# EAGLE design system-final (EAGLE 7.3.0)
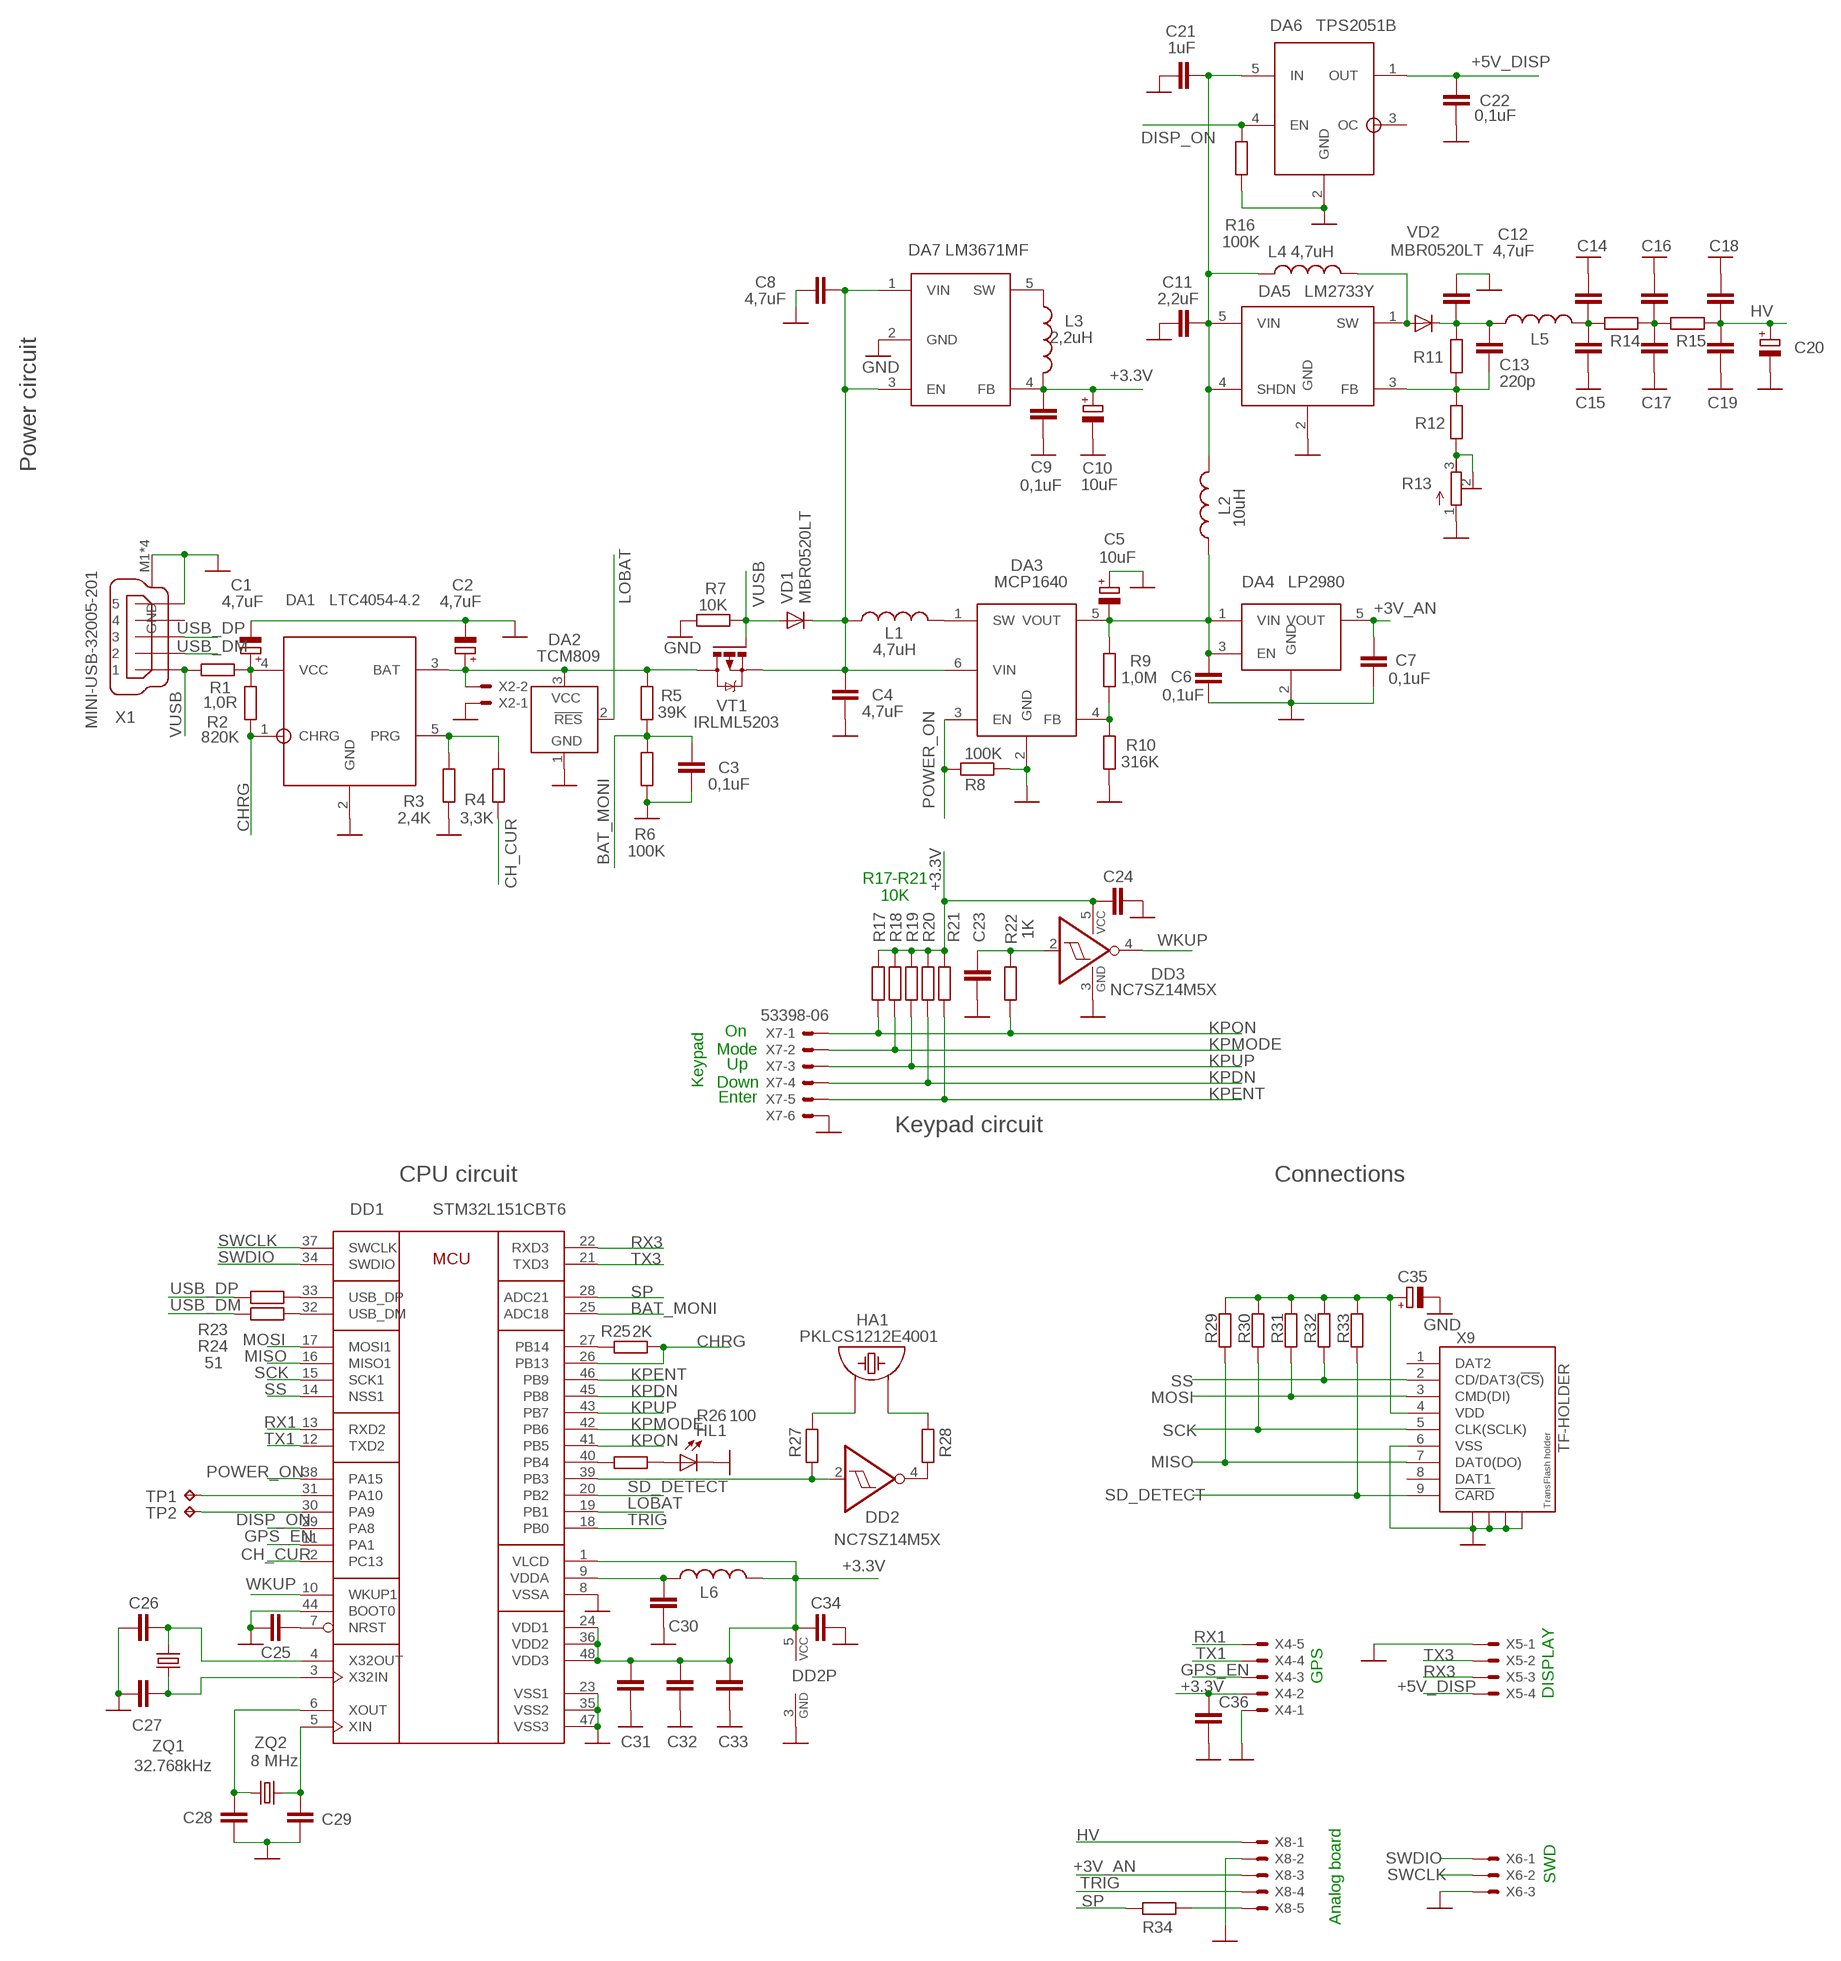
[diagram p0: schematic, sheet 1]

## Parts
C1  4,7uF  CPOL-EUSMCA  [SMC_A]
C2  4,7uF  CPOL-EUSMCA  [SMC_A]
C3  0,1uF  C-EUC0603  [C0603]
C4  4,7uF  C-EUC0805  [C0805]
C5  10uF  CPOL-EUSMCB  [SMC_B]
C6  0,1uF  C-EUC0603  [C0603]
C7  0,1uF  C-EUC0603  [C0603]
C8  4,7uF  C-EUC1206  [C1206]
C9  0,1uF  C-EUC1206  [C1206]
C10  10uF  CPOL-EUSMCB  [SMC_B]
C11  2,2uF  C-EUC0805  [C0805]
C12  4,7uF  C-EUC1206  [C1206]
C13  220p  C-EUC0603  [C0603]
C14  C-EUC0603  [C0603]
C15  C-EUC0603  [C0603]
C16  C-EUC0603  [C0603]
C17  C-EUC0603  [C0603]
C18  C-EUC0603  [C0603]
C19  C-EUC0603  [C0603]
C20  CPOL-EUSMCE  [SMC_E]
C21  1uF  C-EUC0805  [C0805]
C22  0,1uF  C-EUC0805  [C0805]
C23  C-EUC0603  [C0603]
C24  C-EUC0603  [C0603]
C25  C-EUC0603  [C0603]
C26  C-EUC0603  [C0603]
C27  C-EUC0603  [C0603]
C28  C-EUC0603  [C0603]
C29  C-EUC0603  [C0603]
C30  C-EUC0603  [C0603]
C31  C-EUC0603  [C0603]
C32  C-EUC0603  [C0603]
C33  C-EUC0603  [C0603]
C34  C-EUC0603  [C0603]
C35  CPOL-EUSMCA  [SMC_A]
C36  C-EUC0805  [C0805]
DA1  LTC4054-4.2  [SOT23-5L]
DA2  TCM809  [SOT23B-3]
DA3  MCP1640  [SOT23-6]
DA4  LP2980  [SOT23-5L]
DA5  LM2731Y  [SOT23-5L]
DA6  TPS2051B  [SOT23-5L]
DA7  LM3671  [SOT23-5]
DD1  STM32L151CBT6  STM32L151C  [LQFP48]
DD2  NC7SZ14M5X  [SOT23-5]
DD3  NC7SZ14M5X  [SOT23-5]
HA1  PKLCS1212E4001  [PKLCS1212E4001]
HL1  LEDCHIP-LED0805  [CHIP-LED0805]
L1  4,7uH  L-USL1812  [L1812]
L2  10uH  L-USL2825P  [L2825P]
L3  2,2uH  L-USL2825P  [L2825P]
L4  4,7uH  L-USL1812  [L1812]
L5  L-USL2825P  [L2825P]
L6  L-USL3225M  [L3225M]
R1  1,0R  R-EU_M1206  [M1206]
R2  820K  R-EU_R0603  [R0603]
R3  2,4K  R-EU_R0603  [R0603]
R4  3,3K  R-EU_R0603  [R0603]
R5  39K  R-EU_R0603  [R0603]
R6  100K  R-EU_R0603  [R0603]
R7  10K  R-EU_R0603  [R0603]
R8  100K  R-EU_R0603  [R0603]
R9  1,0M  R-EU_R0603  [R0603]
R10  316K  R-EU_R0603  [R0603]
R11  R-EU_R0603  [R0603]
R12  R-EU_R0603  [R0603]
R13  R-TRIMM3103  [RTRIM3103]
R14  R-EU_R0603  [R0603]
R15  R-EU_R0603  [R0603]
R16  100K  R-EU_R0603  [R0603]
R17  10K  R-EU_R0603  [R0603]
R18  10K  R-EU_R0603  [R0603]
R19  10K  R-EU_R0603  [R0603]
R20  10K  R-EU_R0603  [R0603]
R21  10K  R-EU_R0603  [R0603]
R22  1K  R-EU_R0603  [R0603]
R23  51  R-EU_R0603  [R0603]
R24  51  R-EU_R0603  [R0603]
R25  2K  R-EU_R0603  [R0603]
R26  100  R-EU_R0603  [R0603]
R27  R-EU_R0603  [R0603]
R28  R-EU_R0603  [R0603]
R29  R-EU_R0603  [R0603]
R30  R-EU_R0603  [R0603]
R31  R-EU_R0603  [R0603]
R32  R-EU_R0603  [R0603]
R33  R-EU_R0603  [R0603]
R34  R-EU_R0603  [R0603]
TP1  TPB1,27  [B1,27]
TP2  TPB1,27  [B1,27]
VD1  MBR0520LT  [SOD123]
VD2  MBR0520LT  [SOD123]
VT1  IRLML5203  [MICRO3]
X1  MINI-USB-32005-201  [32005-201]
X2  53398-02  [53398-02]
X4  53398-05  [53398-05]
X5  53398-04  [53398-04]
X6  53398-03  [53398-03]
X7  53398-06  [53398-06]
X8  53398-05  [53398-05]
X9  TF-HOLDER  [TF-PULL]
ZQ1  32.768kHz  CRYSTAL-32.768KHZPTH-2X6-KIT  [CRYSTAL-PTH-2X6-CYL-KIT]
ZQ2  CRYSTALPTH-HC49US  [HC49US]

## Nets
5V_D: C11.2 C21.2 DA5.4(SHDN) DA5.5(VIN) DA6.5(IN) L2.2 L4.1
+3.3V: C9.2 C10.+ C24.1 C31.1 C32.1 C33.1 C34.1 C35.+ C36.1 DA7.4(FB) DD1.1(VLCD) DD1.24(VDD1) DD1.36(VDD2) DD1.48(VDD3) DD2.5(VCC) DD3.5(VCC) L3.2 L6.2 R17.2 R18.2 R19.2 R20.2 R21.2 R29.2 R30.2 R31.2 R32.2 R33.2 X4.2 X9.4(VDD)
+3V_AN: C7.1 DA4.5(VOUT) X8.3
+5V_DIRT: C5.- C6.1 DA3.5(VOUT) DA4.1(VIN) DA4.3(EN) L2.1 R9.2
+5V_DISP: C22.1 DA6.1(OUT) X5.4
BAT_MONI: C3.1 DD1.25(ADC18) R5.1 R6.2
BUZ: DD1.39(PB3) DD2.2(I) R27.1
CH_CUR: DD1.2(PC13) R4.1
CHRG: DA1.1(CHRG) DD1.26(PB13) R2.1 R25.1
DISP_ON: DA6.4(EN) DD1.29(PA8) R16.2
GND: C1.- C2.- C3.2 C4.2 C5.+ C6.2 C7.2 C8.1 C9.1 C10.- C11.1 C12.1 C14.1 C15.2 C16.1 C17.2 C18.1 C19.2 C20.- C21.1 C22.2 C23.2 C24.2 C25.2 C26.1 C27.1 C28.2 C29.2 C30.1 C31.2 C32.2 C33.2 C34.2 C35.- C36.2 DA1.2(GND) DA2.1(GND) DA3.2(GND) DA4.2(GND) DA5.2(GND) DA6.2(GND) DA7.2(GND) DD1.8(VSSA) DD1.23(VSS1) DD1.35(VSS2) DD1.44(BOOT0) DD1.47(VSS3) DD2.3(GND) DD3.3(GND) HL1.C R3.1 R6.1 R7.1 R8.1 R10.1 R13.1(A) R16.1 X1.5 X1.M1(GND) X1.M2(GND) X1.M3(GND) X1.M4(GND) X2.1 X4.1 X5.1 X6.3 X7.6 X8.2 X9.6(VSS) X9.S1 X9.S2 X9.S3 X9.S4
GPS_EN: DD1.11(PA1) X4.3
HV: C18.2 C19.1 C20.+ R15.2 X8.1
KPDN: DD1.45(PB8) R20.1 X7.4
KPENT: DD1.46(PB9) R21.1 X7.5
KPMODE: DD1.42(PB6) R18.1 X7.2
KPON: DD1.41(PB5) R17.1 R22.2 X7.1
KPUP: DD1.43(PB7) R19.1 X7.3
LED: DD1.40(PB4) R26.2
LOBAT: DA2.2(!RES) DD1.19(PB1)
MISO: DD1.16(MISO1) R29.1 X9.7(DAT0(DO))
MOSI: DD1.17(MOSI1) R31.1 X9.3(CMD(DI))
N$1: DD1.31(PA10) TP1.TP
N$2: C25.1 DD1.7(NRST)
N$3: C1.+ DA1.4(VCC) R1.2 R2.2
N$5: DA3.1(SW) L1.2
N$6: DA5.1(SW) L4.2 VD2.A
N$7: DA3.4(FB) R9.1 R10.2
N$8: C13.2 DA5.3(FB) R11.1 R12.2
N$9: C12.2 C13.1 L5.1 R11.2 VD2.C
N$10: R12.1 R13.2(S) R13.3(E)
N$11: C28.1 DD1.6(XOUT) ZQ2.1
N$12: C14.2 C15.1 L5.2 R14.1
N$13: C16.2 C17.1 R14.2 R15.1
N$14: C27.2 DD1.3(X32IN) ZQ1.2
N$15: C26.2 DD1.4(X32OUT) ZQ1.1
N$16: C29.1 DD1.5(XIN) ZQ2.2
N$18: DD1.30(PA9) TP2.TP
N$19: DD2.4(O) R28.1
N$20: HA1.P$2 R27.2
N$21: HA1.P$1 R28.2
N$23: HL1.A R26.1
N$24: DA7.5(SW) L3.1
N$25: DD1.27(PB14) R25.2
N$26: C23.1 DD3.2(I) R22.1
N$27: DD1.33(USB_DP) R23.1
N$28: DD1.32(USB_DM) R24.1
N$30: DA1.5(PRG) R3.2 R4.2
POWER_ON: DA3.3(EN) DD1.38(PA15) R8.2
RX1: DD1.13(RXD2) X4.5
RX3: DD1.22(RXD3) X5.3
SCK: DD1.15(SCK1) R30.1 X9.5(CLK(SCLK))
SD_DETECT: DD1.20(PB2) R33.1 X9.9(!CARD)
SP: DD1.28(ADC21) R34.2
SP_IN: R34.1 X8.5
SS: DD1.14(NSS1) R32.1 X9.2(CD/DAT3(!CS!))
SWCLK: DD1.37(SWCLK) X6.2
SWDIO: DD1.34(SWDIO) X6.1
TRIG: DD1.18(PB0) X8.4
TX1: DD1.12(TXD2) X4.4
TX3: DD1.21(TXD3) X5.2
USB_DM: R24.2 X1.2
USB_DP: R23.2 X1.3
VBAT: C2.+ DA1.3(BAT) DA2.3(VCC) R5.2 VT1.3(D) X2.2
VDDA: C30.2 DD1.9(VDDA) L6.1
VMASTER: C4.1 C8.2 DA3.6(VIN) DA7.1(VIN) DA7.3(EN) L1.1 VD1.C VT1.2(S)
VUSB: R1.1 R7.2 VD1.A VT1.1(G) X1.1
WKUP: DD1.10(WKUP1) DD3.4(O)
Unconnected: DA6.3(OC) X1.4 X9.1(DAT2) X9.8(DAT1)

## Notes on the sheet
- DA6   TPS2051B
- DA7 LM3671MF
- DA5   LM2733Y
- Power circuit
- DA3
- DA4   LP2980
- DA1   LTC4054-4.2
- TCM809
- R17-R21
  10K
- On
- Mode
- Up
- Keypad | Down
- Enter
- Keypad circuit
- CPU circuit | Connections
- GPS
- DISPLAY
- 8 MHz
- SWD
- Analog board

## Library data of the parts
C1 C2 C5 C10 C20 C35 = resistor:CPOL-EU: POLARIZED CAPACITOR, European symbol
C3 C4 C6-C9 C11-C19 C21-C34 C36 = resistor:C-EU: CAPACITOR, European symbol
DA1 = LTC4054-4.2:LTC4054-4.2
DA2 = telcom:TCM809: POWER SUPPLY MONITOR replacement for Maxim MAX809 and MAX810; MF: MICROCHIP; MPN: TCM809MENB713; OC_FARNELL: 9762744; OC_NEWARK: 96K3998
DA3 = MCP1640:MCP1640; MPN: MCP1640
DA4 = LP2980:LP2980
DA5 = LM2731Y:LM2731Y
DA6 = TPS2051B:TPS2051B: CURRENT-LIMITED, POWER-DISTRIBUTION SWITCH
DA7 = LM3671MF:LM3671
DD1 = stm32L151C:STM32L151C
DD2 DD3 = 74xx-little-de:NC7SZ14: TinyLogic(R) UHS Inverter with Schmitt Trigger Input Source: http://www.fairchildsemi.com/ds/NC/NC7SZ14.pdf
HA1 = PKLCS1212E:PKLCS1212E4001: SMD piezoelectric buzzer 12x12x3 mm, Murata
HL1 = adafruit:LED: LED
L1-L6 = resistor:L-US: INDUCTOR, American symbol
R1-R12 R14-R34 = resistor:R-EU_: RESISTOR, European symbol
R13 = resistor:R-TRIMM: Trimm resistor
TP1 TP2 = testpad:TP: Test pad
VD1 VD2 = diode:MBR0520LT: SCHOTTKY BARRIER RECTIFIER
VT1 = transistor-power:IRLML5203: HEXFET P-Channel Power MOSFET
X1 = con-cypressindustries:MINI-USB-: MINI USB-B Conector Source: www.cypressindustries.com; OC_FARNELL: unknown; OC_NEWARK: unknown
X2 = con-molex:53?-02: CONNECTOR; OC_FARNELL: unknown; OC_NEWARK: unknown
X4 X8 = con-molex:53?-05: CONNECTOR wire to board 1.25 mm (.049 inch) pitch header; OC_FARNELL: 1125354; OC_NEWARK: unknown
X5 = con-molex:53?-04: CONNECTOR wire to board 1.25 mm (.049 inch) pitch header; OC_FARNELL: 1125367; OC_NEWARK: unknown
X6 = con-molex:53?-03: CONNECTOR wire to board 1.25 mm (.049 inch) pitch header; OC_FARNELL: unknown; OC_NEWARK: unknown
X7 = con-molex:53?-06: CONNECTOR wire to board 1.25 mm (.049 inch) pitch header; OC_FARNELL: 1125368; OC_NEWARK: unknown
X9 = sd-mmc:TF-HOLDER: TF / Micro SD socket is PUSH-PUSH type, the card can be pushed into and auto locked and pushed out by simply press the card. Surface Mounting type.
ZQ1 = SparkFun-Clocks:CRYSTAL-32.768KHZ: 32.768kHz Crystal; PROD_ID: XTAL-10112
ZQ2 = SparkFun-Clocks:CRYSTAL: Crystals (Generic)

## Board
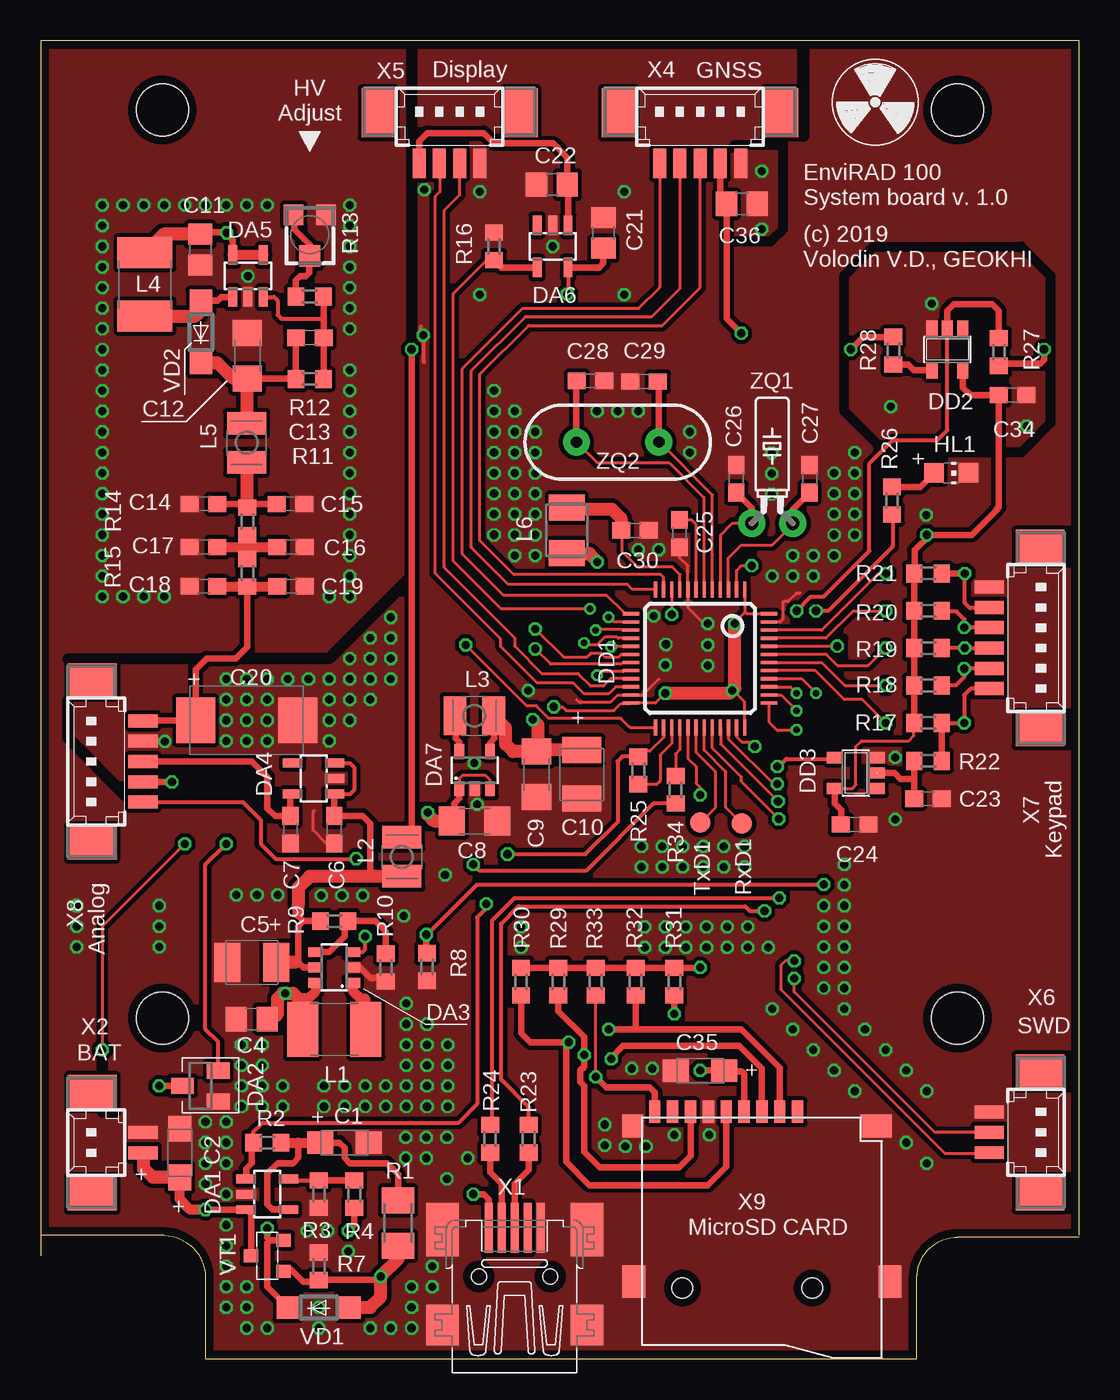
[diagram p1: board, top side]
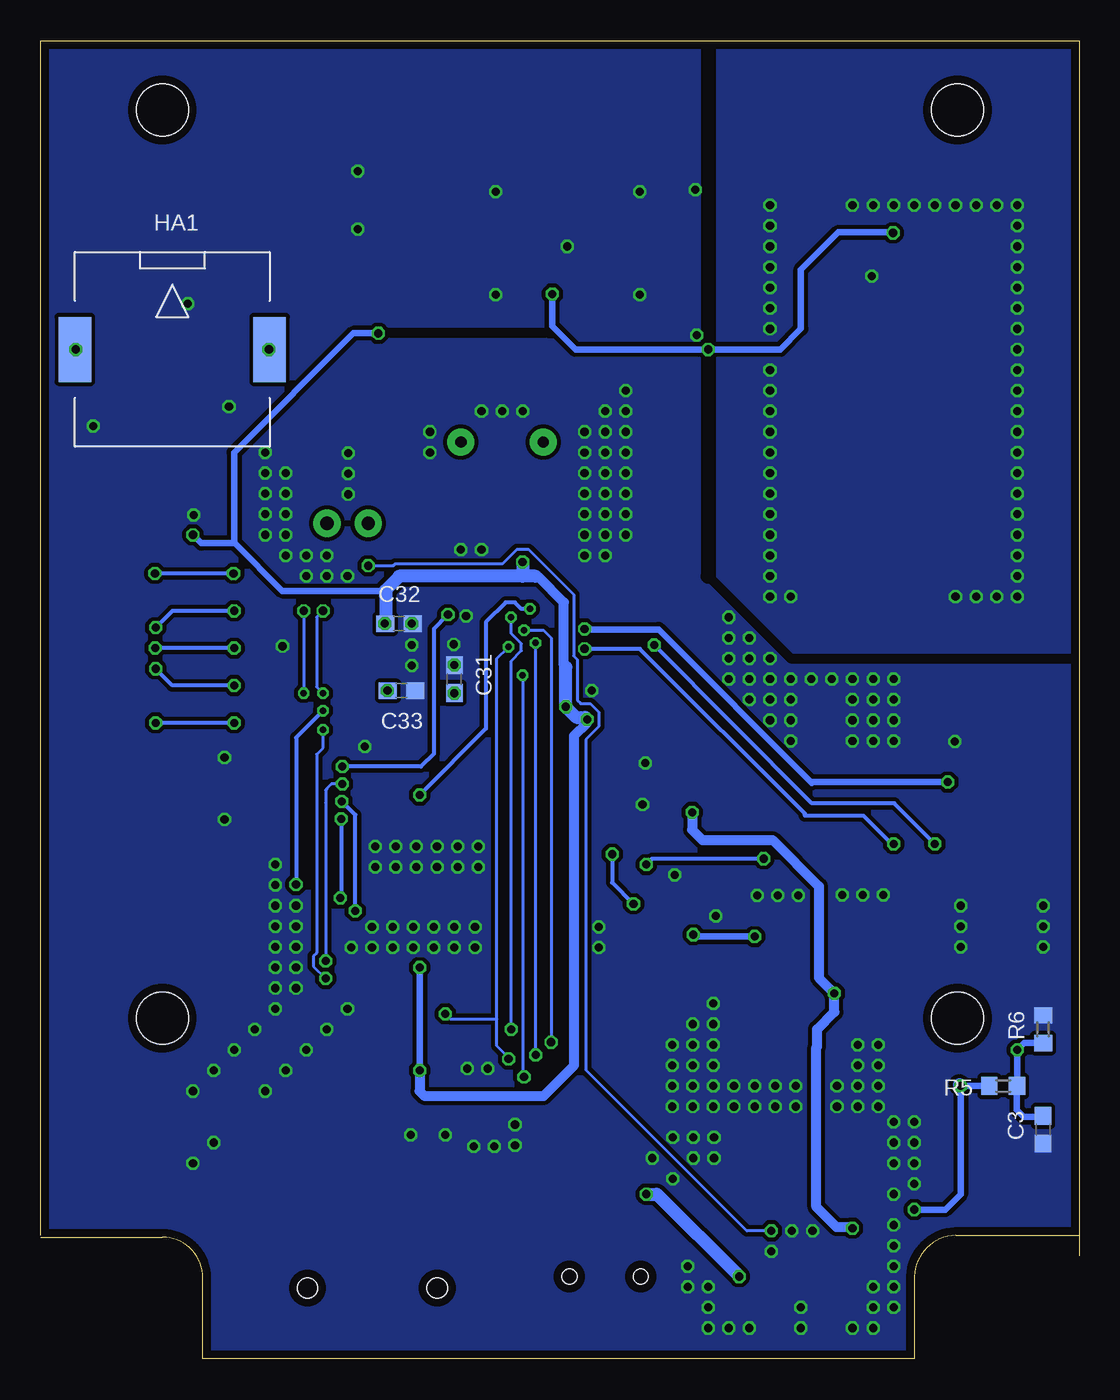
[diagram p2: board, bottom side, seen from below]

Size 64 x 81.27 mm. Coordinates in mm from the lower left corner, seen from the top.
Outline: 53.98,0 10.16,0 10.16,5.08 arc86 7.62,7.62 0,7.62
Outline: 64,7.62 64,81.27 0,81.27 0,7.62
Outline: 54,0 54,5 arc-90 56.5,7.5 64,7.5
Outline: 0,7.62 0,6.35
Copper layers (1*16): Top 0.035mm / dielectric 1.6mm / Bottom 0.035mm
Design rules "Elecrow_2-layer_PCB_eagle_rule": minimum track width 6mil, minimum drill 12mil, track to track 6mil, track to pad 6mil, pad to pad 6mil, via to via 8mil, smd to smd 0mil, copper to edge 20mil, drill to drill 10mil, minimum pad ring 6mil, minimum via ring 6mil, stop-mask expansion 0mil, vias tented up to drill 100mil, thermal gap 10mil
Holes 3.2 mm at 56.5,21 7.5,21 56.5,76.98 7.5,76.98
tRestrict: area 43.2,37.1 to 44.8,38.4; area 48.3,43.2 to 49.5,44.5; 25 lines
bRestrict: 7 lines

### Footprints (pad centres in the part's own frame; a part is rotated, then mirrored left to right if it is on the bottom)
SMC_A = smd 1.6 x 1.4: + -1.5,0; - 1.5,0
C0603 = smd 1.1 x 1: 1 -0.85,0; 2 0.85,0
C0805 = smd 1.3 x 1.5: 1 -0.95,0; 2 0.95,0
SMC_B = smd 1.6 x 2.4: + -1.5,0; - 1.5,0
C1206 = smd 1.6 x 1.8: 1 -1.4,0; 2 1.4,0
SMC_E = smd 2.4 x 2.8: + -3.15,0; - 3.15,0
SOT23-5L = smd 0.55 x 1.2: 1 -0.95,-1.3; 2 0,-1.3; 3 0.95,-1.3; 4 0.95,1.3; 5 -0.95,1.3
SOT23B-3 = smd 1 x 1.4: 1 -0.95,-1.1; 2 0.95,-1.1; 3 0,1.1
SOT23-6 = smd 0.6 x 0.9: 1 -0.95,-1.15; 2 0,-1.15; 3 0.95,-1.15; 4 0.95,1.15; 5 0,1.15; 6 -0.95,1.15
SOT23-5 = smd 0.6 x 0.9: 1 -0.95,-1.15; 2 0,-1.15; 3 0.95,-1.15; 4 0.95,1.15; 5 -0.95,1.15
LQFP48 = smd 0.2 x 1: 1 -2.75,-4.25; 2 -2.25,-4.25; 3 -1.75,-4.25; 4 -1.25,-4.25; 5 -0.75,-4.25; 6 -0.25,-4.25; 7 0.25,-4.25; 8 0.75,-4.25; 9 1.25,-4.25; 10 1.75,-4.25; 11 2.25,-4.25; 12 2.75,-4.25; 25 2.75,4.25; 26 2.25,4.25; 27 1.75,4.25; 28 1.25,4.25; 29 0.75,4.25; 30 0.25,4.25; 31 -0.25,4.25; 32 -0.75,4.25; 33 -1.25,4.25; 34 -1.75,4.25; 35 -2.25,4.25; 36 -2.75,4.25 | smd 1 x 0.2: 13 4.25,-2.75; 14 4.25,-2.25; 15 4.25,-1.75; 16 4.25,-1.25; 17 4.25,-0.75; 18 4.25,-0.25; 19 4.25,0.25; 20 4.25,0.75; 21 4.25,1.25; 22 4.25,1.75; 23 4.25,2.25; 24 4.25,2.75; 37 -4.25,2.75; 38 -4.25,2.25; 39 -4.25,1.75; 40 -4.25,1.25; 41 -4.25,0.75; 42 -4.25,0.25; 43 -4.25,-0.25; 44 -4.25,-0.75; 45 -4.25,-1.25; 46 -4.25,-1.75; 47 -4.25,-2.25; 48 -4.25,-2.75
SOT23-5' = smd 0.69 x 0.99: 1 -0.95,-1.29; 2 0,-1.29; 3 0.95,-1.29; 4 0.95,1.3; 5 -0.95,1.3
PKLCS1212E4001 = smd 2 x 4: P$1 6,0; P$2 -6,0
CHIP-LED0805 = smd 1.2 x 1.2: A 0,-1.05; C 0,1.05
L1812 = smd 1.9 x 3.4: 1 -1.95,0; 2 1.95,0
L2825P = smd 1.4 x 2.4: 1 -1.2,0; 2 1.2,0
L3225M = smd 1.6 x 2.2: 1 -1.4,0; 2 1.4,0
M1206 = smd 1.6 x 2: 1 -1.4,0; 2 1.4,0
R0603 = smd 1 x 1.1: 1 -0.85,0; 2 0.85,0
RTRIM3103 = smd 1.2 x 1.25: 1 -1,-1.225; 3 1,-1.225 | smd 1.3 x 1.3: 2 0,1.3
B1,27 = smd 1.27 x 1.27: TP 0,0
SOD123 = smd 1.4 x 1.4: A 1.9,0; C -1.9,0
MICRO3 = smd 0.8 x 0.9: 1 -0.95,-1; 2 0.95,-1; 3 0,1
32005-201 = smd 3.1 x 0.5: 1 3,1.6; 2 3,0.8; 3 3,0; 4 3,-0.8; 5 3,-1.6 | smd 2.5 x 2: M1 -3,-4.45; M2 -3,4.45 | smd 3.3 x 2: M3 2.9,4.45; M4 2.9,-4.45 | hole 0.9: 0,2.2; 0,-2.2
53398-02 = smd 0.8 x 1.8: 1 0.625,-2.5; 2 -0.625,-2.5 | smd 2.1 x 3: S1 3.125,0.625; S2 -3.125,0.625
53398-05 = smd 0.8 x 1.8: 1 2.5,-2.5; 2 1.25,-2.5; 3 0,-2.5; 4 -1.25,-2.5; 5 -2.5,-2.5 | smd 2.1 x 3: S1 5,0.625; S2 -5,0.625
53398-04 = smd 0.8 x 1.8: 1 1.875,-2.5; 2 0.625,-2.5; 3 -0.625,-2.5; 4 -1.875,-2.5 | smd 2.1 x 3: S1 4.375,0.625; S2 -4.375,0.625
53398-03 = smd 0.8 x 1.8: 1 1.25,-2.5; 2 0,-2.5; 3 -1.25,-2.5 | smd 2.1 x 3: S1 3.75,0.625; S2 -3.75,0.625
53398-06 = smd 0.8 x 1.8: 1 3.125,-2.5; 2 1.875,-2.5; 3 0.625,-2.5; 4 -0.625,-2.5; 5 -1.875,-2.5; 6 -3.125,-2.5 | smd 2.1 x 3: S1 5.625,0.625; S2 -5.625,0.625
TF-PULL = smd 0.7 x 1.4: 1 -2.2,-7.62; 2 -1.1,-7.62; 3 0,-7.62; 4 1.1,-7.62; 5 2.2,-7.62; 6 3.3,-7.62; 7 4.4,-7.62; 8 5.5,-7.62; 9 6.6,-7.62 | smd 1.4 x 2: S1 -7.9,2.85; S2 7.9,2.85 | smd 1.28 x 1.4: S3 7.96,-6.75 | smd 1.95 x 1.4: S4 -7.025,-6.75 | hole 1.25: -3.1,3.25; 4.9,3.25
CRYSTAL-PTH-2X6-CYL-KIT = drill 0.813 pad 1.676: 1 -1.27,0; 2 1.27,0
HC49US = drill 0.7 pad 1.651: 1 -2.54,0; 2 2.54,0

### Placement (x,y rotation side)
C1  18.73,13.34 0 top
C2  8.57,12.7 90 top
C3  2.22,14.13 270 bottom
C4  13.02,20.95 180 top
C5  13.02,24.45 0 top
C6  18.1,32.62 270 top
C7  15.4,32.62 270 top
C8  26.75,33.16 180 top
C9  30.56,36.04 90 top
C10  33.36,36.04 270 top
C11  9.84,68.38 90 top
C12  12.74,61.83 270 top
C13  16.59,62.94 0 top
C14  10.04,52.7 0 top
C15  15.4,52.7 0 top
C16  15.44,50.05 180 top
C17  10.04,50.05 180 top
C18  10.04,47.62 0 top
C19  15.44,47.62 0 top
C20  12.7,39.37 0 top
C21  34.69,69.41 270 top
C22  31.51,72.39 180 top
C23  54.69,34.53 0 top
C24  50.16,32.94 0 top
C25  39.37,50.88 270 top
C26  42.86,54.25 270 top
C27  47.39,54.25 270 top
C28  33.89,60.29 0 top
C29  37.19,60.25 180 top
C30  36.63,51.08 180 top
C31  38.5,41.91 90 bottom
C32  41.91,45.32 0 bottom
C33  41.75,41.2 0 bottom
C34  59.89,59.41 0 top
C35  40.64,17.78 180 top
C36  43.22,71.2 0 top
DA1  13.97,10.16 270 top
DA2  9.84,16.83 90 top
DA3  18.1,24.13 90 top
DA4  16.83,35.78 90 top
DA5  12.78,66.75 0 top
DA6  31.55,68.58 180 top
DA7  26.75,36.29 0 top
DD1  40.64,43.18 180 top
DD2  NC7SZ14M5X  [SOT23-5']  55.88,62.23 180 top
DD3  NC7SZ14M5X  [SOT23-5']  50.24,36.12 90 top
HA1  55.88,62.23 0 bottom
HL1  56.12,54.61 270 top
L1  18.1,20.32 0 top
L2  22.26,30.96 90 top
L3  26.73,39.65 0 top
L4  6.43,66.24 270 top
L5  12.7,56.48 270 top
L6  32.42,51.08 270 top
R1  22.03,8.37 90 top
R2  13.97,13.34 0 top
R3  17.14,10.16 90 top
R4  19.33,10.16 90 top
R5  4.68,16.83 180 bottom
R6  2.22,20.32 270 bottom
R7  17.14,5.71 270 top
R8  23.81,24.17 90 top
R9  18.1,26.99 180 top
R10  21.27,24.13 90 top
R11  16.59,60.4 180 top
R12  16.59,65.48 0 top
R13  16.59,69.29 180 top
R14  12.74,51.63 270 top
R15  12.74,48.46 270 top
R16  27.94,68.58 270 top
R17  54.69,39.21 180 top
R18  54.69,41.51 180 top
R19  54.69,43.81 180 top
R20  54.69,46.12 180 top
R21  54.69,48.42 180 top
R22  54.69,36.87 0 top
R23  30.08,13.57 270 top
R24  27.7,13.57 270 top
R25  36.83,36.27 270 top
R26  52.47,52.9 270 top
R27  59.05,62.07 270 top
R28  52.55,62.15 90 top
R29  31.91,23.26 90 top
R30  29.61,23.26 90 top
R31  39.05,23.26 90 top
R32  36.67,23.26 90 top
R33  34.21,23.26 90 top
R34  39.13,35.08 90 top
TP1  43.22,33 0 top
TP2  40.65,33.06 0 top
VD1  17.14,3.17 0 top
VD2  9.88,63.3 90 top
VT1  13.97,6.35 90 top
X1  29.21,5.08 90 top
X2  3.81,13.34 90 top
X4  40.64,76.2 0 top
X5  25.2,76.2 0 top
X6  60.96,13.97 270 top
X7  60.96,44.45 270 top
X8  3.81,36.83 90 top
X9  44.45,7.62 180 top
ZQ1  45.09,51.51 0 top
ZQ2  35.56,56.52 0 top

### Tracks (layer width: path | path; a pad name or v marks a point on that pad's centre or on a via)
5V_D  (via drill 0.5)
  Top 0.254: DA6.5 32.5,65.68 v32.46,65.64 | 22.86,32.75 L2.2
  Top 0.406: DA6.5 34.42,67.28 34.69,67.55 C21.2 | v22.86,62.23 22.86,32.75 | DA5.5 11.83,68.97 11.51,69.29 11.51,69.41 v11.47,69.41 11.47,69.45 9.96,69.45 C11.2
  Top 0.61: DA5.4 DA5.5
  Top 0.813: C11.2 7.57,69.33 L4.1
  Bottom 0.406: v32.46,65.64 32.46,63.67 31.03,62.23 v22.86,62.23 18.41,62.23 17.14,63.5 17.14,67.15 14.84,69.45 11.51,69.45 v11.47,69.41
+3.3V  (via drill 0.5)
  Top 0.2: v38.5,41.04 37.89,40.43 DD1.24 36.36,40.4 35.76,40.4 35.32,39.97 32.38,39.97 32.15,40.2 v31.63,40.2 | v42.78,45.32 42.78,45.4 43.42,46.04 | 43.42,46.04 43.42,47.4 DD1.1 | DD1.48 43.53,45.93 43.42,46.04 | DD1.36 43.39,40.51 42.66,41.23 | DD3.5 50.01,35.17 50.24,35.4 50.24,37.74 50.6,38.1 53.5,38.1 53.82,38.42 53.82,39.19 R17.2
  Top 0.406: R17.2 R18.2 R19.2 R20.2 R21.2 53.86,48.44 53.86,49.85 54.81,50.8 | R30.2 R29.2 R33.2 R32.2 R31.2 40.62,24.11 v40.64,24.13 | X9.4 43.35,17.57 43.18,17.74 42.18,17.74 C35.+ v40.64,17.78 | DD2.5 56.83,59.89 57.31,59.41 C34.1 59.05,59.4 59.05,52.51 58.86,52.31 58.86,52.27 57.39,50.8 54.81,50.8 | X4.2 41.89,71.58 C36.1 42.27,64.13 v43.18,63.22 | DD3.5 48.94,34.24 49.33,33.85 49.33,32.96 C24.1 | 54.81,50.8 v54.61,50.8 | DA7.4 27.7,37.98 27.96,38.24 27.96,39.62 L3.2
  Top 0.813: v38.5,41.04 42.47,41.04 v42.62,41.2 42.66,41.23 42.78,41.35 v42.78,45.32 | L6.2 32.45,49.65 33.81,49.65 34.3,49.16 v34.3,49.13 | C10.+ 30.66,37.54 | 30.66,37.54 C9.2 29.12,37.44 28.65,37.9 28.65,38.9 L3.2 | 30.66,37.54 30.66,39.09 v30.32,39.43
  Bottom 0.2: v38.5,41.04 C31.1 | C32.1 v42.78,45.32
  Bottom 0.406: v40.64,24.13 v40.64,17.78 | v43.18,63.22 44.73,63.22 52.07,55.88 52.07,50.32 52.03,50.28 | 52.03,50.28 49.09,47.35 43.06,47.35 42.74,47.03 | 52.03,50.28 54.09,50.28 v54.61,50.8 | 42.76,41.33 v42.62,41.2
  Bottom 0.61: v30.32,39.43 30.32,39.21 31.11,38.42 31.11,18.1 33.02,16.19 40.32,16.19 40.64,16.51 v40.64,17.78 | 31.63,42.62 31.75,42.74 31.75,46.63 33.38,48.26 33.51,48.26
  Bottom 0.813: 42.7,45.4 v42.78,45.32 | 33.51,48.26 34.29,48.26 | 34.29,48.26 41.91,48.26 41.91,48.22 42.74,47.39 42.74,47.03 42.74,45.4 42.86,45.28 | v30.32,39.43 30.44,39.55 30.98,39.55 v31.63,40.2 31.63,42.62 | v34.3,49.13 34.3,48.27 34.29,48.26 | v42.62,41.2 C33.1
+3V_AN
  Top 0.406: X8.3 13.01,36.83 13.97,35.87 13.97,33.93 14.45,33.46 15.38,33.46 C7.1 15.4,34.7 DA4.5
+5V_DIRT
  Top 0.254: DA4.3 19.05,36.73 19.33,36.45 19.33,35.08 19.05,34.81 18.15,34.81 DA4.1
  Top 0.406: DA3.5 16.19,24.13 15.88,24.45 | 15.88,24.45 15.88,26.67 16.19,26.99 | 16.19,26.99 R9.2 | 15.88,24.45 15.72,24.45 | 13.97,24.45 C5.- | 20.32,29.76 20.32,33.02 19.87,33.47 C6.1 | 15.88,27.46 15.88,27.3 16.19,26.99 | C6.1 18.1,34.8 DA4.1 | C6.1
  Top 0.7: 15.88,27.74 15.88,27.46
  Top 0.75: 15.88,27.98 15.88,27.74
  Top 0.813: 15.72,24.45 C5.- | L2.1 20.32,29.76 16.58,29.76 15.88,29.05 15.88,27.98
+5V_DISP
  Top 0.406: X5.4 23.33,75.08 23.81,75.56 27.3,75.56 27.94,74.93 31.59,74.93 32.46,74.06 C22.1 32.5,72.35 DA6.1
BAT_MONI  (via drill 0.5)
  Top 0.2: v8.89,31.75 3.81,26.67 v3.81,19.05 | DD1.25 36.31,38.93 35.76,39.49 31.32,39.49 30.52,40.28 29.92,40.28 v26.19,44.01
  Bottom 0.254: v8.89,31.75 11.39,34.25 16.47,34.25 v26.19,44.01
  Bottom 0.406: R6.2 3.39,19.47 v3.81,19.05 3.81,16.85 R5.1 3.83,15.34 3.41,14.92 2.28,14.92 C3.1
BUZ  (via drill 0.4, 0.5)
  Top 0.2: DD1.39 46.2,41.43 v46.59,41.04
  Top 0.254: v46.59,46.12 47.47,46.99 48.26,46.99 51.08,49.81 51.08,55.2 52.51,56.63 55.24,56.63 55.88,57.27 DD2.2
  Top 0.406: DD2.2 55.88,64.61 56.28,65.01 58.66,65.01 59.05,64.61 R27.1
  Bottom 0.2: v46.59,46.12 46.99,45.72 46.99,41.43 v46.59,41.04
CH_CUR  (via drill 0.5)
  Top 0.2: DD1.2 42.89,48.6 43.18,48.9 v43.81,48.9
  Top 0.406: R4.1 19.33,8.26 v18.97,7.9
  Bottom 0.2: v43.81,48.9 42.27,48.9 42.15,49.01 35.54,49.01 34.67,49.89 33.91,49.89 31.16,47.13 31.16,43.34 30.92,43.1 30.92,40.6 30.71,40.4 30.12,40.4 29.61,39.89 29.61,38.97 30.4,38.18 30.4,17.82 20.48,7.9 v18.97,7.9
CHRG  (via drill 0.5)
  Top 0.2: DD1.26 38.39,38.29 38.37,38.29 37.54,37.47 37.17,37.47 R25.1
  Top 0.254: R25.1 35.85,37.12 35.56,36.83 35.56,33.1 33.58,31.11 v28.77,31.11 | R2.1 13.12,13.99 13.69,14.56 25.76,14.56 26.91,15.72 26.91,27.23 27.46,27.78 v27.46,28.06
  Top 0.406: DA1.1 12.67,11.72 13.02,12.06 13.02,13.23 R2.1
  Bottom 0.254: v28.77,31.11 28.77,29.37 v27.46,28.06
DISP_ON  (via drill 0.4, 0.5)
  Top 0.2: DD1.29 39.89,37.02 40.4,36.51 40.4,35.48 40.64,35.24 v40.64,34.77 | v33.85,46.24 28.38,46.24 25.44,49.17 25.44,65.68 27.46,67.71
  Top 0.254: 27.46,67.71 27.92,67.71 R16.2
  Top 0.406: DA6.4 28.39,67.28 R16.2
  Bottom 0.254: v40.64,34.77 36.55,38.85 36.55,45.42 35.34,46.63 34.77,46.63 34.37,46.24 v33.85,46.24
GND  (via drill 0.5)
  Top 0.2: C32.2 40.88,45.32 39.89,46.31 39.89,46.32 DD1.8 | DD1.47 44.9,45.44 45.6,45.44 45.76,45.6 45.76,46.67 45.8,46.71 46.08,46.71 46.59,47.23 46.81,47.23 | DD1.44 v49.09,43.93 | DD1.23 37.12,40.93 38.1,41.91 | v44.01,37.74 43.74,38.02 43.22,38.02 42.89,38.35 DD1.35 | 39.89,47.31 39.89,48.9 39.37,49.41 C25.2 | 33.02,40.64 33.18,40.48 35.12,40.48 35.56,40.92 36.47,40.92 | C6.2 17.62,31.77 16.79,32.6 16.79,33.73 16.85,33.73 16.85,33.81 | 18.28,35.8 DA4.2
  Top 0.254: 23.61,61.48 23.61,62.98 23.42,63.18 23.42,63.62 23.45,63.66
  Top 0.406: DA3.2 19.68,24.13 20.32,23.5 21.06,23.5 | 41.27,15.32 41.2,15.24
  other vias: 16.43,7.9 17.7,7.9 11.43,10.16 11.43,12.06 11.43,13.34 11.43,14.61 12.38,15.56 13.65,15.56 14.92,15.56 22.54,15.56 12.38,16.83 13.65,16.83 14.92,16.83 17.46,15.56 18.73,15.56 20,15.56 21.27,15.56 17.46,16.83 18.73,16.83 20,16.83 21.27,16.83 22.5,13.65 22.5,12.38 10.16,13.34 10.16,12.06 10.16,14.61 10.16,10.79 11.43,8.26 11.43,6.99 11.43,5.71 12.7,4.45 12.7,3.17 12.7,1.91 22.86,1.91 21.59,1.91 13.97,1.91 24.13,4.45 13.65,18.1 13.65,19.37 12.38,19.37 7.3,27.94 7.3,26.67 12.78,66.75 34.77,14.45 34.77,13.18 36.04,13.1 39.05,13.81 38.5,42.78 41.2,13.81 48.26,27.94 49.53,29.21 49.53,30.48 54.57,52.03 52.67,37.07 36.43,17.9 31.55,68.58 45.05,53.3 45.05,54.57 45.05,55.84 7.66,38.06 29.61,26.63 29.61,25.36 37.23,26.63 37.23,25.36 38.5,26.63 39.77,26.63 41.04,26.63 42.31,26.63 43.58,26.63 37.03,30.32 38.3,30.32 39.57,30.32 40.84,30.32 42.11,30.32 43.38,30.32 48.26,26.67 48.26,25.4 48.26,24.13 48.26,22.86 49.53,21.59 50.8,20.32 44.85,25.36 41.12,45.32 19.05,67.31 19.05,66.04 19.05,64.77 19.05,63.5 19.05,60.96 19.05,58.42 19.05,57.15 19.05,55.88 19.05,54.61 19.05,53.34 19.05,52.07 19.05,50.8 19.05,49.53 19.05,48.26 17.78,46.99 3.81,46.99 3.81,48.26 3.81,49.53 3.81,50.8 3.81,52.07 3.81,53.34 3.81,54.61 3.81,55.88 3.81,57.15 3.81,58.42 3.81,60.96 3.81,62.23 3.81,63.5 3.81,64.77 3.81,66.04 3.81,67.31 3.81,68.58 3.81,69.85 3.81,71.12 6.35,71.12 5.08,71.12 7.62,71.12 8.89,71.12 10.16,71.12 11.43,71.12 12.7,71.12 13.97,71.12 3.81,59.69 5.08,46.99 19.05,46.99 19.05,71.12 7.3,25.4 18.57,28.57 19.84,28.57 12.38,18.1 23.77,13.65 23.77,12.38 24.13,5.71 11.43,4.45 11.43,3.17 25.04,13.65 25.04,11.11 22.54,16.83 23.81,15.56 25.08,15.56 23.81,16.83 17.14,3.17 17.14,1.91 20.32,1.91 37.31,13.1 37.03,31.59 38.3,31.59 39.57,31.59 40.84,31.59 42.11,31.59 43.38,31.59 38.5,25.36 39.77,25.36 41.04,25.36 42.31,25.36 43.58,25.36 49.53,27.94 49.53,26.67 49.53,25.4 49.53,22.86 49.53,24.13 19.05,68.58 19.05,69.85 2.22,27.94 2.22,26.67 2.22,25.4 37.7,17.9 41.12,44.01 22.54,18.1 22.54,19.37 22.54,20.64 23.81,20.64 23.81,18.1 23.81,19.37 25.08,16.83 25.08,18.1 25.08,19.37 17.3,28.57 22.38,27.3 22.54,21.91 44.45,69.65 44.45,73.22 34.29,58.42 36.83,58.42 35.56,58.42 41.12,42.74 38.54,44.05 37.78,45.8 27.07,71.95 54.93,65.05 60.76,57.51 52.39,58.7 19.05,59.69 27.94,52.07 27.94,50.8 52.67,33.26 17.78,41.91 16.51,41.91 15.24,41.91 13.97,41.91 12.7,41.91 11.43,41.91 11.43,40.64 12.7,40.64 13.97,40.64 11.43,39.37 12.7,39.37 13.97,39.37 11.43,38.1 12.7,38.1 13.97,38.1 19.05,43.18 20.32,44.45 21.59,45.72 21.59,44.45 20.32,43.18 19.05,41.91 20.32,41.91 21.59,43.18 21.59,41.91 17.78,40.64 19.05,40.64 30.04,41.2 23.65,72.07 27.07,65.6 35.96,65.6 35.96,71.95 23.57,63.1 14.61,28.61 13.34,28.61 12.06,28.61 24.92,29.84 18.97,6.63 29.21,49.53 30.48,49.53 36.83,49.89 38.1,49.89 26.31,12.38 22.86,3.17 22.86,4.45 50.16,16.51 45.09,21.59 46.35,20.32 47.62,19.05 48.9,17.78 52.07,19.05 53.34,17.78 29.21,50.8 27.94,53.34 27.94,54.61 27.94,55.88 40.01,57.15 40.01,55.88 30.48,57.15 30.48,55.88 54.61,16.51 54.61,12.06 53.34,13.34 29.21,52.07 29.21,53.34 29.21,54.61 27.94,57.15 30.48,50.8 30.48,52.07 30.48,53.34 29.21,55.88 30.48,54.61 46.35,49.53 47.62,49.53 48.9,49.53 45.09,48.26 46.35,48.26 47.62,48.26 48.9,50.8 48.9,52.07 50.16,50.8 50.16,52.07 50.16,53.34 17.78,39.37 20.32,40.64 19.05,39.37 17.78,38.1 29.21,57.15 27.94,58.42 27.94,59.69 29.21,58.42 50.16,54.61 48.9,53.34 50.16,55.88 48.9,54.61 6.35,46.99 7.62,46.99 26.73,36.73 26.91,34.17
  pour Top (isolate 0.254, no thermals): 0,0 64.14,0 64.14,81.28 0,81.28
  pour Bottom (isolate 0.254, no thermals): 0,81.28 63.5,81.28 63.5,0 0,0
GPS_EN
  Top 0.2: DD1.11 38.39,48.17 38.22,48.34 29.16,48.34 27.07,50.44 27.07,60.7 30.07,63.7 38.3,63.7 40.64,66.04 X4.3
HV
  Top 0.406: X8.1 6.35,39.37 C20.+ 9.55,42.49 10.24,43.18 12.03,43.18 12.74,43.89 R15.2
  Top 0.61: C18.2 C19.1 14.57,47.61 R15.2
KPDN  (via drill 0.5)
  Top 0.2: v52.07,46.12 50.09,46.12 48.4,44.43 DD1.45
  Top 0.254: X7.4 56.92,45.08 | 56.92,45.08 v56.91,45.09 | 56.92,45.08 56.92,45.59 56.43,46.08 55.58,46.08 R20.1
  Bottom 0.254: v52.07,46.12 55.88,46.12 v56.91,45.09
KPENT  (via drill 0.5)
  Top 0.2: DD1.46 48.15,44.93 51.63,48.42 v52.11,48.42
  Top 0.254: 58.41,46.28 57.27,46.28 56.95,46.59 v56.95,48.42
  Top 0.406: 58.41,46.28 X7.5 | v56.95,48.42 R21.1
  Bottom 0.254: v52.11,48.42 v56.95,48.42
KPMODE  (via drill 0.5)
  Top 0.2: DD1.42 48.15,42.93 49.57,41.51 v52.07,41.51
  Top 0.254: X7.2 56.94,42.58 v56.91,42.55 56.91,42.03 56.4,41.51 R18.1
  Bottom 0.254: v52.07,41.51 55.88,41.51 v56.91,42.55
KPON  (via drill 0.5)
  Top 0.2: v52.07,39.21 50.64,40.64 49.53,40.64 47.74,42.43 DD1.41
  Top 0.254: R17.1 v56.91,39.21 56.91,40.92 57.32,41.33 X7.1
  Top 0.406: R17.1 R22.2
  Bottom 0.254: v52.07,39.21 v56.91,39.21
KPUP  (via drill 0.5)
  Top 0.2: v52.07,43.81 51,42.74 50.99,42.76 49.09,42.76 48.42,43.43 DD1.43
  Top 0.254: X7.3 v56.94,43.83 55.55,43.83 R19.1
  Bottom 0.254: 52.08,43.83 v56.94,43.83
  Bottom 0.406: 52.08,43.83 v52.07,43.81
LED  (via drill 0.4, 0.5)
  Top 0.2: DD1.40 46.89,41.93 v47.78,41.04
  Top 0.254: R26.2 52.51,52.01 52.51,50.09 48.54,46.12 v47.78,46.12
  Bottom 0.2: v47.78,46.12 v47.78,41.04
LOBAT  (via drill 0.5)
  Top 0.2: DD1.19 35.87,42.93 35.76,42.82 31.43,42.82 v30.48,43.77
  Top 0.254: DA2.2 10.94,19.54 10.16,20.32 10.16,30.48 v11.43,31.75
  Bottom 0.254: v11.43,31.75 11.55,31.75 13.29,33.5 16.91,33.5 16.91,33.62 27.07,43.77 v30.48,43.77
MISO  (via drill 0.4, 0.5)
  Top 0.2: v33.5,44.13 33.58,44.05 34.37,44.05 34.37,44.09 34.81,44.53 35.48,44.53 35.58,44.43 DD1.16
  Top 0.406: X9.7 40.05,12.51 39.37,11.83 34.45,11.83 33.5,12.78 33.5,16.83 33.26,17.07 33.26,17.78 33.5,18.02 v33.5,18.73 33.5,19.84 31.91,21.43 R29.1
  Bottom 0.2: v33.5,18.73 v33.5,44.13
MOSI  (via drill 0.4, 0.5)
  Top 0.2: DD1.17 35.2,43.93 v35.16,43.89
  Top 0.406: X9.3 44.45,17.9 43.06,19.29 35.88,19.29 35.16,18.57 v35.16,18.49 | v39.05,21.27 R31.1
  Bottom 0.2: v35.16,18.49 35.16,18.57 35.88,19.29 35.88,20.95 | 35.88,20.95 35.88,43.18 v35.16,43.89 | v39.05,21.27 38.73,20.95 35.88,20.95
N$1
  Top 0.2: TP1.TP 42.23,33.99 42.23,36.2 40.89,37.53 DD1.31
N$2
  Top 0.2: DD1.7 40.39,51.45 40.12,51.71 39.39,51.71 C25.1
N$3
  Top 0.406: DA1.4 14.29,9.21 13.97,9.53 13.97,11.43 14.61,12.06 15.56,12.06 15.88,12.38 15.88,13.34 | C1.+ 18.41,13.34 18.73,13.02 18.73,12.38 19.05,12.06 21.35,12.06 22.03,11.39 R1.2
  Top 0.61: R2.2 15.88,13.34 C1.+
N$5
  Top 0.61: DA3.1 19.25,22.66 19.68,22.23 20,22.23 20,20.36 L1.2
N$6
  Top 0.406: DA5.1 11.12,65.45 10.91,65.25 9.93,65.25 VD2.A
  Top 0.813: L4.2 9.56,64.29 9.72,64.45 9.72,65.04 VD2.A
N$7
  Top 0.406: R10.2 21.27,26.35 20.64,26.99 R9.1 18.73,26.77 18.73,26.04 17.78,25.08 DA3.4
N$8
  Top 0.254: DA5.3 14.4,65.45 14.61,65.25 14.61,64.37 14.84,64.14 17.36,64.14 17.44,64.21
  Top 0.406: R11.1 C13.2 17.44,64.21 R12.2
N$9
  Top 0.406: C12.2 15.71,60.43 R11.2 C13.1
  Top 0.813: VD2.C 10.91,61.4 11.88,60.43 C12.2 12.71,60.4 L5.1
N$10
  Top 0.406: R12.1 15.74,66.5 15.99,66.75 16.35,66.75 16.55,66.95 16.55,67.95 R13.2 16.59,68.7 15.64,69.65 15.64,70.47 R13.3
N$11
  Top 0.2: DD1.6 40.88,47.44 40.88,53.1 38.73,55.24 34.29,55.24 ZQ2.1
  Top 0.406: C28.1 33.02,60.26 ZQ2.1
N$12
  Top 0.406: C14.2 12.74,52.7 | 12.74,52.7 C15.1 | R14.1 12.74,52.7
  Top 0.813: 12.74,52.7 12.74,55.24 L5.2
N$13
  Top 0.61: R14.2 12.74,50.05 | 12.74,50.05 R15.1 12.74,49.23 | C17.1 12.74,50.05 | 12.74,50.05 C16.2
N$14
  Top 0.2: DD1.3 42.39,49.38 43.18,50.16 45.09,50.16 46.35,51.44 ZQ1.2
  Top 0.406: C27.2 46.35,52.37 ZQ1.2
N$15
  Top 0.2: DD1.4 41.89,50.22 41.91,50.24 41.91,50.8 42.62,51.51 ZQ1.1
  Top 0.406: C26.2 43.81,52.45 ZQ1.1
N$16
  Top 0.2: DD1.5 41.39,49.57 41.39,53.26 38.14,56.52 ZQ2.2
  Top 0.406: C29.1 38.1,60.18 ZQ2.2
N$18
  Top 0.2: TP2.TP 41.59,34 41.59,36.2 40.39,37.4 DD1.30
N$19
  Top 0.406: R28.1 53.48,61.3 53.82,60.96 54.9,60.96 DD2.4
N$20  (via drill 0.5)
  Top 0.406: v61.83,62.23 61.83,61.59 61.59,61.36 59.19,61.36 R27.2
  Bottom 0.2: v61.83,62.23 HA1.P$2
N$21  (via drill 0.5)
  Top 0.406: R28.2 50.7,63 v49.93,62.23
  Bottom 0.2: HA1.P$1 v49.93,62.23
N$23
  Top 0.406: HL1.A 54.21,53.75 R26.1
N$24
  Top 0.406: DA7.5 25.8,38.04 25.6,38.24 25.6,39.64 L3.1
N$25
  Top 0.2: DD1.27 38.89,37.94 38.18,37.23 38.18,35.64 37.94,35.4 36.85,35.4 R25.2
N$26
  Top 0.406: R22.1 53.84,35.8 | 53.84,35.8 C23.1 | DD3.2 52.63,36.12 52.98,35.76 53.8,35.76 53.84,35.8
N$27  (via drill 0.5)
  Top 0.2: DD1.33 41.91,38.91 41.91,37.9 v45.44,34.37
  Top 0.254: R23.1 30.08,15.52 28.38,17.22 28.38,26.83 29.45,27.9 43.42,27.9 43.7,27.62 v44.61,27.62
  Bottom 0.254: v44.61,27.62 44.61,33.54 v45.44,34.37
N$28  (via drill 0.5)
  Top 0.2: DD1.32 41.39,37.67 43.18,35.88 43.18,35.6 v45.48,33.3
  Top 0.254: R24.1 27.82,14.54 27.82,27.03 29.21,28.42 v45.52,28.42
  Bottom 0.254: v45.48,33.3 45.48,28.46 v45.52,28.42
N$30
  Top 0.254: DA1.5 15.37,11.01 R3.2
  Top 0.406: R3.2 R4.2
POWER_ON  (via drill 0.4, 0.5)
  Top 0.2: DD1.38 44.9,40.92 45.64,40.92 v46.59,39.97
  Top 0.254: DA3.3 19.84,25.08 20,25.24 v20,26.04 | v48.26,29.25 26.91,29.25 23.81,26.15 v23.77,26.15
  Top 0.406: R8.2 23.77,25.06 v23.77,26.15
  Bottom 0.254: v46.59,39.97 48.26,38.3 v48.26,29.25
  Bottom 0.406: v23.77,26.15 23.65,26.04 v20,26.04
RX1
  Top 0.2: X4.5 38.14,66.04 36.87,64.77 29.72,64.77 26,61.05 26,49.61 28.54,47.07 34.88,47.07 35.98,45.97 35.98,45.93 DD1.13
RX3
  Top 0.2: DD1.22 35.44,41.43 35,41 33.5,41 32.82,41.67 30.6,41.67 28.36,43.91 28.36,44.39 24.33,48.42 24.33,71.68 24.61,71.95 24.61,73.67
  Top 0.254: 24.61,73.67 X5.3
SCK  (via drill 0.4, 0.5)
  Top 0.2: v34.21,44.93 34.25,44.97 35.8,44.97 35.83,44.93 DD1.15
  Top 0.406: X9.5 42.25,11.85 41.12,10.72 33.81,10.72 32.38,12.14 32.38,19.37 v32.54,19.53 30.16,19.53 29.61,20.08 R30.1
  Bottom 0.2: v34.21,44.93 33.02,44.93 32.54,44.45 v32.54,19.53
SD_DETECT  (via drill 0.4, 0.5)
  Top 0.2: v34.21,17.38 R33.1 | DD1.20 35.94,42.43 35.88,42.37 34.51,42.37 v34.29,42.15
  Top 0.406: X9.9 37.85,16.44 37.54,16.75 34.85,16.75 v34.21,17.38
  Bottom 0.2: v34.29,42.15 34.29,17.46 v34.21,17.38
SP
  Top 0.2: 38.92,35.93 R34.2 39.13,37.31 39.39,37.56 DD1.28
SP_IN  (via drill 0.5)
  Top 0.254: R34.1 37.77,34.23 33.62,30.08 27.07,30.08 v26.67,30.48 | X8.5 6.35,34.29 12.5,34.29 13.57,33.22 13.57,31.75 14.49,30.84 v19.45,30.84
  Bottom 0.254: v19.45,30.84 26.31,30.84 v26.67,30.48
SS  (via drill 0.4, 0.5)
  Top 0.2: DD1.14 35.29,45.43 v35,45.72
  Top 0.406: X9.2 45.55,17.94 43.17,20.32 36.83,20.32 | 36.83,20.32 v35,20.32 | R32.1 36.67,20.48 36.83,20.32
  Bottom 0.2: v35,20.32 35,43.02 34.37,43.66 34.37,44.09 35,44.73 v35,45.72
SWCLK  (via drill 0.4, 0.5)
  Top 0.2: X6.2 55.09,13.97 46.43,22.62 v46.43,23.45 | v46.59,38.77 46.55,38.73 45.4,38.73 44.89,39.25 DD1.37
  Bottom 0.2: v46.43,23.45 47.19,24.21 47.19,24.84 46.99,25.04 46.99,37.27 46.59,37.66 v46.59,38.77
SWDIO  (via drill 0.5)
  Top 0.2: DD1.34 42.39,38.22 45.16,35.44 v45.4,35.44 | v46.43,24.53 45.88,24.53 45.6,24.25 45.6,22.78 55.72,12.66 58.4,12.66 X6.1
  Bottom 0.2: v45.4,35.44 46.08,35.44 46.35,35.16 46.35,35.12 46.43,35.04 46.43,34.29 46.43,24.61 v46.43,24.53
TRIG  (via drill 0.5)
  Top 0.2: DD1.18 35.77,43.43 35.58,43.24 34.79,43.24 34.53,43.5 33.89,43.5 33.66,43.26 32.23,43.26 v30.48,45.01
  Top 0.406: X8.4 8.08,35.58 v8.1,35.56
  Bottom 0.2: v30.48,45.01 30.48,44.97
  Bottom 0.406: 30.48,44.97 25.92,44.97 16.47,35.52 16.43,35.56 v8.1,35.56
TX1
  Top 0.2: DD1.12 36.47,47.43 36.16,47.74 28.83,47.74 26.55,50.02 26.55,60.91 29.89,64.25 37.66,64.25 39.41,66 39.41,73.68 X4.4
TX3
  Top 0.2: DD1.21 35.14,41.93 34.69,41.47 33.89,41.47 33.14,42.23 30.92,42.23 29.21,43.93 29.21,44.45 24.88,48.78 24.88,70.8 25.84,71.75 X5.2
  Top 0.254: 25.88,73.65 X5.2
USB_DM
  Top 0.406: X1.2 28.41,10.8 27.7,11.51 R24.2
USB_DP
  Top 0.406: X1.3 29.21,10.79 30.08,11.67 R23.2
VBAT  (via drill 0.5)
  Top 0.406: v10.16,9.21 DA1.3 | v7.3,16.83 DA2.3 | 6.35,12.67 X2.2 | DA1.3 13.06,9.21 | VT1.3 12.97,8.91 DA1.3
  Top 0.61: v10.16,9.21 9.21,9.21 8.57,9.84 C2.+
  Top 0.813: C2.+ 6.9,11.2 6.35,11.75 6.35,12.67
  Bottom 0.406: v10.16,9.21 8.26,9.21 7.3,10.16 v7.3,16.83 R5.2
  Bottom 0.813: 7.38,16.91 v7.3,16.83
VDDA
  Top 0.2: DD1.9 39.39,48.36 38.93,48.82 36.79,48.82 35.84,49.77 35.84,51.02 C30.2
  Top 0.61: 35.84,51.13 C30.2
  Top 0.813: L6.1 32.52,52.39 35.2,52.39 35.78,51.81 C30.2
VMASTER  (via drill 0.5)
  Top 0.2: DA7.3 27.7,35.7 27.44,35.96 25.98,35.96 25.8,35.78 DA7.1
  Top 0.406: 13.97,4.45 VD1.C | 13.97,4.45 13.96,4.45 | VT1.2 14.13,7.3 | 14.13,7.3 13.97,7.46 v13.97,8.06 | 13.97,4.45 13.97,7.14 14.13,7.3 | DA7.1 25.8,34.55 25.48,34.23 25.48,33.19 C8.2
  Top 0.61: DA3.6 16.95,22.66 16.51,22.23 15.88,22.23 15.88,20.59 L1.1
  Top 0.813: C4.1 14.29,20.95 14.61,21.27 14.61,22.23 14.92,22.54 v15.08,22.54 15.56,22.54 15.88,22.23 | v23.85,33.7 23.85,33.56 24.23,33.18 C8.2
  Bottom 0.61: v23.85,33.7 23.85,32.62 23.22,31.99 18.89,31.99 16.03,29.13 16.03,23.5 v15.08,22.54 15.08,21.39 L1.1 16.15,19.25 16.19,19.21 16.19,9.37 14.96,8.14 14.05,8.14 v13.97,8.06
VUSB  (via drill 0.5)
  Top 0.254: 27.62,9.36 27.62,8.09 X1.1
  Top 0.406: VT1.1 15.07,5.5 15.46,5.5 16.19,4.76 17.04,4.76 R7.2 20.74,4.87 v20.95,5.08 | 27.62,9.36 27.62,9.84 27.3,10.16 v26.67,10.16
  Top 0.813: VD1.A 20.32,3.17 20.95,3.81 v20.95,5.08 22.03,6.15 R1.1
  Bottom 0.813: v26.67,10.16 26.04,10.16 v20.95,5.08
WKUP  (via drill 0.5)
  Top 0.2: DD1.10 v38.89,45.88
  Top 0.254: v38.89,45.88 | v45.4,36.51 45.48,36.51 45.96,36.99 48.87,36.99 DD3.4
  Bottom 0.254: v45.4,36.51 40.56,36.51 39.77,37.31 39.77,45.01 v38.89,45.88

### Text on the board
tPlace: EnviRAD 100 / System board v. 1.0 | (c) 2019 / Volodin V.D., GEOKHI | + | + | + | + | + | + | +
tNames: Display | GNSS | HV / Adjust | Keypad | TxD1 | RxD1 | Analog | SWD | BAT | MicroSD CARD
bNames: HA1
